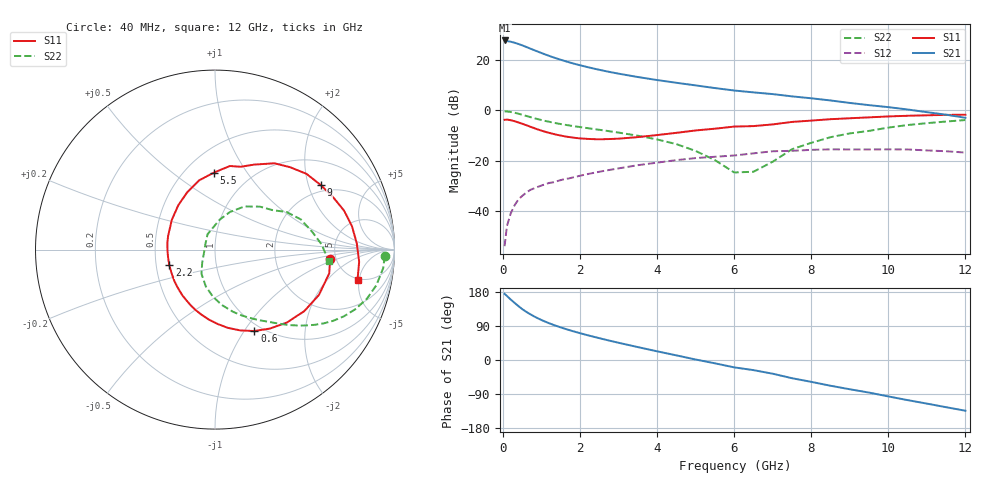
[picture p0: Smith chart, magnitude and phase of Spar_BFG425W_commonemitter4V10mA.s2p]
! Filename: 410bfg425.001
! BFG425W Field C1
! V1=8.334E-001V,V2=4.000E+000V, I1=1.119E-004A, I2=1.001E-002A
# GHz  S  MA  R 50
!  S11  S21  S12  S22
!Freq(GHz)  Mag  Ang  Mag  Ang  Mag  Ang  Mag  Ang
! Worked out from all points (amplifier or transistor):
!   44 points, 40 MHz to 12 GHz, reference 50 ohm
!   highest |S21| = 27.7 dB at 40 MHz (marker M1)
!   |S21| within 3 dB of that: start of sweep to 670 MHz
!   unconditionally stable (mu >= 1): start of sweep to 42.69 MHz; 1.875 GHz to end of sweep
!   at 700 MHz: K = 0.55, MSG = 28.1 dB, |S12| = -31.7 dB
!   at 2.4 GHz: K = 1.10, MAG = 18.7 dB, |S12| = -24.7 dB
!   at 12 GHz: K = 1.40, MAG = 3.1 dB, |S12| = -16.8 dB
!   S11 on the Smith chart (normalised r, x): 40 MHz: 4.48, -0.78; 600 MHz: 0.92, -1.11; 2.2 GHz: 0.59, -0.11; 5.5 GHz: 0.68, +0.72; 9 GHz: 1.77, +2.42; 12 GHz: 4.78, -4.77
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0.04  0.644 -4.5  24.18 174.5  0.002 47.8  0.946 -2.2
0.2  0.632 -23.5  22.83 159.4  0.009 70.8  0.921 -12.4
0.3  0.604 -34.6  21.76 150.6  0.013 68.2  0.889 -18.0
0.4  0.571 -45.3  20.58 142.2  0.017 64.7  0.85 -23.0
0.5  0.536 -55.1  19.32 134.1  0.02 61.5  0.809 -27.3
0.6  0.504 -64.2  17.99 127.3  0.023 58.9  0.769 -31.1
0.8  0.442 -80.6  15.61 115.4  0.028 54.6  0.696 -37.0
0.9  0.415 -87.9  14.55 110.2  0.03 53.1  0.664 -39.5
1  0.392 -94.9  13.58 105.4  0.032 51.9  0.636 -41.7
1.2  0.354 -107.8  11.92 96.8  0.036 49.7  0.588 -45.7
1.4  0.324 -119.7  10.56 89.4  0.039 48.2  0.547 -49.0
1.6  0.302 -131.1  9.462 82.6  0.043 46.8  0.514 -52.1
2.2  0.269 -161.4  7.126 65.3  0.054 42.7  0.439 -61.3
3  0.272 163.9  5.3 45.4  0.07 35.7  0.359 -74.1
3.5  0.292 145.6  4.545 34.0  0.081 30.3  0.311 -82.9
4.5  0.355 115.8  3.494 12.2  0.102 17.4  0.212 -103.9
5.5  0.429 90.8  2.744 -8.8  0.119 2.9  0.102 -134.4
6.5  0.483 72.8  2.254 -26.7  0.139 -8.1  0.06 155.6
8.5  0.662 39.6  1.558 -68.0  0.167 -44.9  0.291 55.7
9  0.691 31.2  1.391 -77.2  0.166 -53.2  0.346 43.8
10.5  0.774 9.8  1.032 -105.9  0.166 -80.5  0.507 19.4
12  0.812 -12.1  0.706 -133.9  0.144 -111.1  0.637 -5.8
